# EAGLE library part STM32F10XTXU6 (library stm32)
STM32F101/103 36pad VFQPFN36
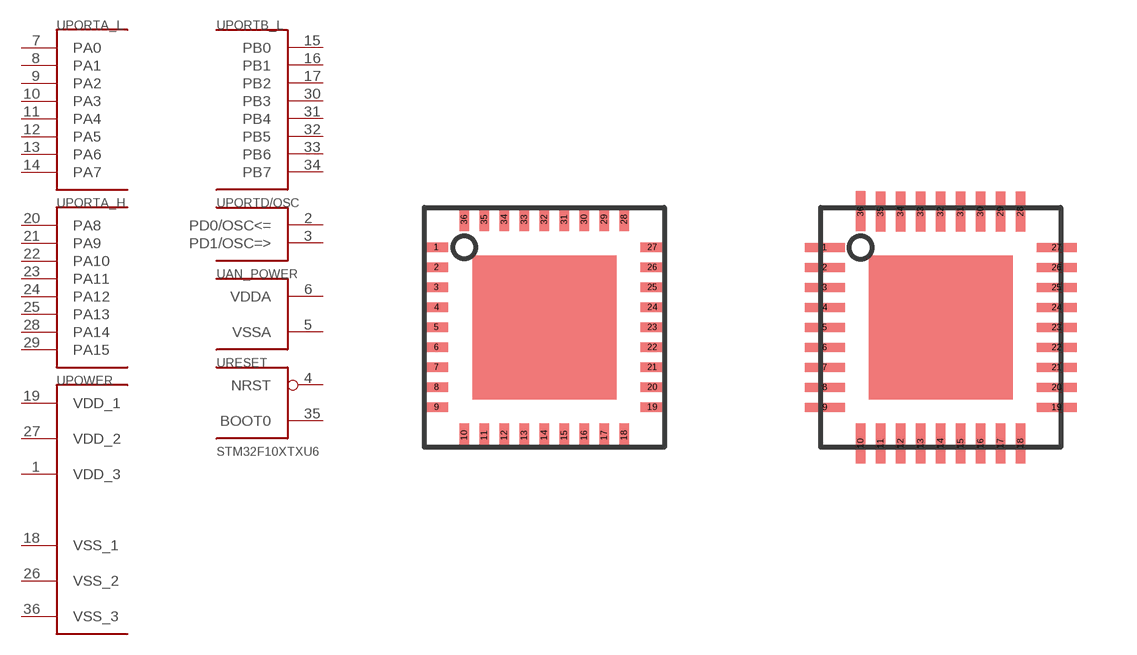
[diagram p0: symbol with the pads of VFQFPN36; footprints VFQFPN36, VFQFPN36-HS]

Designator prefix U; gates PORTA_L=PORT_A_L PORTA_H=PORT_A_H PORTB_L=PORT_B_L POWER=VCC_VDD_S PORTD/OSC=PORT_D_2 AN_POWER=BAT_AN_S RESET=BOOT_RST

## STM32F10XTXU6  [VFQFPN36]
1  POWER:VDD_3  pwr
2  PORTD/OSC:PD0/OSC<=
3  PORTD/OSC:PD1/OSC=>
4  RESET:NRST  in
5  AN_POWER:VSSA  pwr
6  AN_POWER:VDDA  pwr
7  PORTA_L:PA0
8  PORTA_L:PA1
9  PORTA_L:PA2
10  PORTA_L:PA3
11  PORTA_L:PA4
12  PORTA_L:PA5
13  PORTA_L:PA6
14  PORTA_L:PA7
15  PORTB_L:PB0
16  PORTB_L:PB1
17  PORTB_L:PB2
18  POWER:VSS_1  pwr
19  POWER:VDD_1  pwr
20  PORTA_H:PA8
21  PORTA_H:PA9
22  PORTA_H:PA10
23  PORTA_H:PA11
24  PORTA_H:PA12
25  PORTA_H:PA13
26  POWER:VSS_2  pwr
27  POWER:VDD_2  pwr
28  PORTA_H:PA14
29  PORTA_H:PA15
30  PORTB_L:PB3
31  PORTB_L:PB4
32  PORTB_L:PB5
33  PORTB_L:PB6
34  PORTB_L:PB7
35  RESET:BOOT0  in
36  POWER:VSS_3  pwr

## STM32F10XTXU6HS  [VFQFPN36-HS]
Pads as for VFQFPN36

## Footprint VFQFPN36 (pad centres in mm)
36 contact QFN 0.5mm pin space
smd 0.6 x 0.23: 1 -2.7,2; 2 -2.7,1.5; 3 -2.7,1; 4 -2.7,0.5; 5 -2.7,0; 6 -2.7,-0.5; 7 -2.7,-1; 8 -2.7,-1.5; 9 -2.7,-2; 19 2.7,-2; 20 2.7,-1.5; 21 2.7,-1; 22 2.7,-0.5; 23 2.7,0; 24 2.7,0.5; 25 2.7,1; 26 2.7,1.5; 27 2.7,2
smd 0.23 x 0.6: 10 -2,-2.7; 11 -1.5,-2.7; 12 -1,-2.7; 13 -0.5,-2.7; 14 0,-2.7; 15 0.5,-2.7; 16 1,-2.7; 17 1.5,-2.7; 18 2,-2.7; 28 2,2.7; 29 1.5,2.7; 30 1,2.7; 31 0.5,2.7; 32 0,2.7; 33 -0.5,2.7; 34 -1,2.7; 35 -1.5,2.7; 36 -2,2.7

## Footprint VFQFPN36-HS (pad centres in mm)
VFQFPN36 with 0.3mm extended tracks to aid hand soldering.
smd 1 x 0.23: 1 -2.9,2; 2 -2.9,1.5; 3 -2.9,1; 4 -2.9,0.5; 5 -2.9,0; 6 -2.9,-0.5; 7 -2.9,-1; 8 -2.9,-1.5; 9 -2.9,-2; 19 2.9,-2; 20 2.9,-1.5; 21 2.9,-1; 22 2.9,-0.5; 23 2.9,0; 24 2.9,0.5; 25 2.9,1; 26 2.9,1.5; 27 2.9,2
smd 0.23 x 1: 10 -2,-2.9; 11 -1.5,-2.9; 12 -1,-2.9; 13 -0.5,-2.9; 14 0,-2.9; 15 0.5,-2.9; 16 1,-2.9; 17 1.5,-2.9; 18 2,-2.9; 28 2,2.9; 29 1.5,2.9; 30 1,2.9; 31 0.5,2.9; 32 0,2.9; 33 -0.5,2.9; 34 -1,2.9; 35 -1.5,2.9; 36 -2,2.905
